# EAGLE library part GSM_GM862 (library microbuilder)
GM862 Cellular Module with GPS Proven layout and schematic for GM862 cellular module with SiRF III GPS. Spark Fun Electronics SKU : CEL-07917 Footprint taken from the Sparkfun Eagle library (CC-SA license).
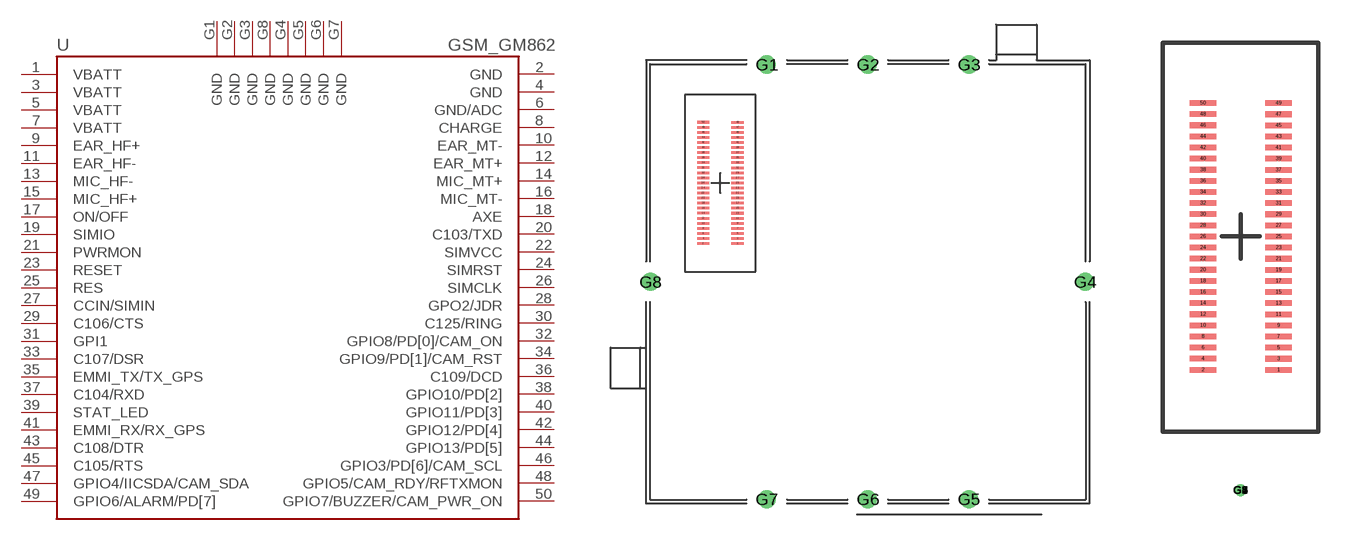
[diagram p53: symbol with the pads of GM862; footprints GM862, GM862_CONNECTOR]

Designator prefix U

## GSM_GM862GND  [GM862]
1  VBATT  pwr
2  GND  pwr
3  VBATT  pwr
4  GND  pwr
5  VBATT  pwr
6  GND/ADC  pwr
7  VBATT  pwr
8  CHARGE  in
9  EAR_HF+  out
10  EAR_MT-  out
11  EAR_HF-  out
12  EAR_MT+  out
13  MIC_HF-  in
14  MIC_MT+  in
15  MIC_HF+  in
16  MIC_MT-  in
17  ON/OFF  in
18  AXE  in
19  SIMIO
20  C103/TXD  in
21  PWRMON  out
22  SIMVCC  pwr
23  RESET  in
24  SIMRST  out
25  RES
26  SIMCLK  out
27  CCIN/SIMIN
28  GPO2/JDR  out
29  C106/CTS
30  C125/RING  out
31  GPI1  in
32  GPIO8/PD[0]/CAM_ON
33  C107/DSR  out
34  GPIO9/PD[1]/CAM_RST
35  EMMI_TX/TX_GPS  out
36  C109/DCD  out
37  C104/RXD  out
38  GPIO10/PD[2]
39  STAT_LED  out
40  GPIO11/PD[3]
41  EMMI_RX/RX_GPS  in
42  GPIO12/PD[4]
43  C108/DTR  in
44  GPIO13/PD[5]
45  C105/RTS  in
46  GPIO3/PD[6]/CAM_SCL
47  GPIO4/IICSDA/CAM_SDA
48  GPIO5/CAM_RDY/RFTXMON
49  GPIO6/ALARM/PD[7]
50  GPIO7/BUZZER/CAM_PWR_ON
G1  GND  pwr
G2  GND  pwr
G3  GND  pwr
G4  GND  pwr
G5  GND  pwr
G6  GND  pwr
G7  GND  pwr
G8  GND  pwr

## GSM_GM862GM862_CONNECTOR  [GM862_CONNECTOR]
Pads as for GM862

## Footprint GM862 (pad centres in mm)
smd 1.2 x 0.25: 1 -12.898,3.791; 2 -16.298,3.794; 3 -12.898,4.291; 4 -16.298,4.294; 5 -12.898,4.791; 6 -16.298,4.794; 7 -12.898,5.291; 8 -16.298,5.294; 9 -12.898,5.791; 10 -16.298,5.794; 11 -12.899,6.29; 12 -16.298,6.294; 13 -12.898,6.791; 14 -16.298,6.794; 15 -12.898,7.291; 16 -16.298,7.294; 17 -12.898,7.791; 18 -16.298,7.794; 19 -12.898,8.291; 20 -16.298,8.294; 21 -12.898,8.791; 22 -16.298,8.794; 23 -12.898,9.291; 24 -16.298,9.294; 25 -12.898,9.791; 26 -16.298,9.794; 27 -12.898,10.291; 28 -16.298,10.294; 29 -12.898,10.791; 30 -16.298,10.794; 31 -12.898,11.291; 32 -16.298,11.294; 33 -12.898,11.791; 34 -16.298,11.794; 35 -12.898,12.291; 36 -16.298,12.294; 37 -12.898,12.791; 38 -16.298,12.794; 39 -12.898,13.291; 40 -16.298,13.294; 41 -12.898,13.791; 42 -16.298,13.794; 43 -12.898,14.291; 44 -16.298,14.294; 45 -12.898,14.791; 46 -16.298,14.794; 47 -12.898,15.291; 48 -16.298,15.294; 49 -12.898,15.791; 50 -16.298,15.794
drill 1.2: G1 -10,21.5; G2 0,21.5; G3 10,21.5; G4 21.5,0; G5 10,-21.5; G6 0,-21.5; G7 -10,-21.5; G8 -21.5,0

## Footprint GM862_CONNECTOR (pad centres in mm)
smd 1.2 x 0.25: 1 1.707,-6.016; 2 -1.693,-6.013; 3 1.707,-5.516; 4 -1.693,-5.513; 5 1.707,-5.016; 6 -1.693,-5.013; 7 1.707,-4.516; 8 -1.693,-4.513; 9 1.707,-4.016; 10 -1.693,-4.013; 11 1.706,-3.517; 12 -1.693,-3.513; 13 1.707,-3.016; 14 -1.693,-3.013; 15 1.707,-2.516; 16 -1.693,-2.513; 17 1.707,-2.016; 18 -1.693,-2.013; 19 1.707,-1.516; 20 -1.693,-1.513; 21 1.707,-1.016; 22 -1.693,-1.013; 23 1.707,-0.516; 24 -1.693,-0.513; 25 1.707,-0.016; 26 -1.693,-0.013; 27 1.707,0.484; 28 -1.693,0.487; 29 1.707,0.984; 30 -1.693,0.987; 31 1.707,1.484; 32 -1.693,1.487; 33 1.707,1.984; 34 -1.693,1.987; 35 1.707,2.484; 36 -1.693,2.487; 37 1.707,2.984; 38 -1.693,2.987; 39 1.707,3.484; 40 -1.693,3.487; 41 1.707,3.984; 42 -1.693,3.987; 43 1.707,4.484; 44 -1.693,4.487; 45 1.707,4.984; 46 -1.693,4.987; 47 1.707,5.484; 48 -1.693,5.487; 49 1.707,5.984; 50 -1.693,5.987
drill 0.025 pad 0.025: G1 0,-11.43; G2 0,-11.43; G3 0,-11.43; G4 0,-11.43; G5 0,-11.43; G6 0,-11.43; G7 0,-11.43; G8 0,-11.43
